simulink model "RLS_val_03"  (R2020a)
settings: Solver=ode45  StartTime=0.0  StopTime=1000  RelTol=1e-3  EnableMultiTasking=on
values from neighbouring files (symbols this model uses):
  Ts = 0.05    [init_model.m]
libraries: ctrlSharedLib x2

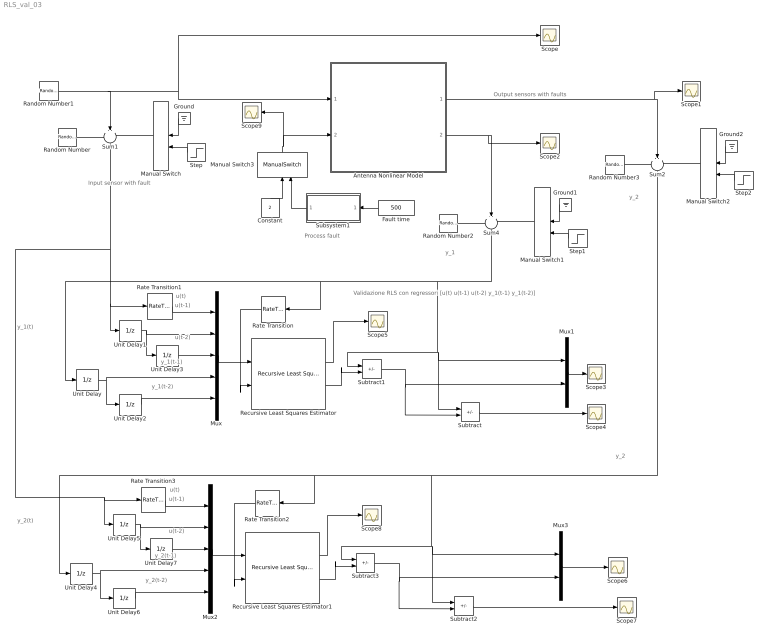
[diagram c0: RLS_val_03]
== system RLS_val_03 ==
  note: Validazione RLS con regressori [u(t) u(t-1) u(t-2) y_1(t-1) y_1(t-2)]
  note: y_1(t)
  note: y_1(t-1)
  note: y_2
  note: y_1
  note: u(t)
  note: Output sensors with faults
  note: Process fault
  note: Input sensor with fault
  note: u(t-1)
  note: y_1(t-2)
  note: u(t-2)
  note: u(t-1)
  note: y_2(t)
  note: y_2(t-1)
  note: y_2
  note: y_2(t-2)
  note: u(t-2)
  note: u(t)
  Antenna Nonlinear Model : Subsystem
  Constant : Constant  Value=2
  Fault time : Constant  Value=500
  Ground : Ground
  Ground1 : Ground
  Ground2 : Ground
  Manual Switch{,1..3} (4 alike) : ManualSwitch
  Mux : Mux  Inputs=5
  Mux1 : Mux  Inputs=2
  Mux2 : Mux  Inputs=5
  Mux3 : Mux  Inputs=2
  Random Number : RandomNumber  Variance=0.0001  Seed=1  SampleTime=Ts
  Random Number1 : RandomNumber  Variance=0.1  SampleTime=10
  Random Number2 : RandomNumber  Variance=0.00001  Seed=2  SampleTime=Ts
  Random Number3 : RandomNumber  Variance=0.00001  Seed=3  SampleTime=Ts
  Rate Transition{,1..3} (4 alike) : RateTransition  OutPortSampleTime=Ts
  Recursive Least Squares Estimator : ctrlSharedLib/Recursive Least Squares Estimator  InitialEstimateSource=None  InitialParameterData=5  P0=1e4  InitialRegressors=0  InitialOutputs=0  History=Infinite  WindowLength=200  EstimationMethod=Forgetting Factor  AdaptationParameter=1  HasTimeVaryingAdaptationParameter=off  NormalizationBias=eps  OutputError=on  OutputP=off  AddEnablePort=off  InputProcessing=Sample-based  Ts=Ts
  Recursive Least Squares Estimator1 : ctrlSharedLib/Recursive Least Squares Estimator  InitialEstimateSource=None  InitialParameterData=5  P0=1e4  InitialRegressors=0  InitialOutputs=0  History=Infinite  WindowLength=200  EstimationMethod=Forgetting Factor  AdaptationParameter=1  HasTimeVaryingAdaptationParameter=off  NormalizationBias=eps  OutputError=on  OutputP=off  AddEnablePort=off  InputProcessing=Sample-based  Ts=Ts
  Scope{,1..9} (10 alike) : Scope
  Step : Step  Time=500  SampleTime=0
  Step1 : Step  Time=1500  SampleTime=0
  Step2 : Step  Time=500  SampleTime=0
  Subsystem1 : Subsystem
  Subtract{,1..3} (4 alike) : Sum  Inputs=+-
  Sum1 : Sum  Inputs=+++  SaturateOnIntegerOverflow=on
  Sum2 : Sum  Inputs=+++  SaturateOnIntegerOverflow=on
  Sum4 : Sum  Inputs=+++  SaturateOnIntegerOverflow=on
  Unit Delay{,1..7} (8 alike) : UnitDelay  SampleTime=Ts  HasFrameUpgradeWarning=on
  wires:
  Random Number1/1 -> Scope/1, Antenna Nonlinear Model/1(force), Sum1/2
  Random Number/1 -> Sum1/1
  Manual Switch/1 -> Sum1/3
  Ground/1 -> Manual Switch/1
  Step/1 -> Manual Switch/2
  Random Number2/1 -> Sum4/1
  Ground1/1 -> Manual Switch1/1
  Manual Switch1/1 -> Sum4/3
  Step1/1 -> Manual Switch1/2
  Antenna Nonlinear Model/2(velocity) -> Sum4/2, Scope2/1
  Random Number3/1 -> Sum2/1
  Ground2/1 -> Manual Switch2/1
  Manual Switch2/1 -> Sum2/3
  Step2/1 -> Manual Switch2/2
  Antenna Nonlinear Model/1(angle) -> Sum2/2, Scope1/1
  Fault time/1 -> Subsystem1/1(Fault time)
  Subsystem1/1(Fault) -> Manual Switch3/2
  Manual Switch3/1 -> Scope9/1, Antenna Nonlinear Model/2(drag)
  Constant/1 -> Manual Switch3/1
  Mux/1 -> Recursive Least Squares Estimator/1
  Unit Delay/1 -> Mux/4, Unit Delay2/1
  Unit Delay1/1 -> Unit Delay3/1, Mux/2
  Unit Delay3/1 -> Mux/3
  Unit Delay2/1 -> Mux/5
  Subtract1/1 -> Subtract/2, Mux1/2
  Sum4/1 -> Subtract/1, Mux1/1, Subtract1/1, Rate Transition/1, Unit Delay/1
  Subtract/1 -> Scope4/1
  Mux1/1 -> Scope3/1
  Rate Transition/1 -> Recursive Least Squares Estimator/2
  Recursive Least Squares Estimator/2 -> Subtract1/2
  Recursive Least Squares Estimator/1 -> Scope5/1
  Rate Transition1/1 -> Mux/1
  Subtract3/1 -> Subtract2/2, Mux3/2
  Mux2/1 -> Recursive Least Squares Estimator1/1
  Rate Transition2/1 -> Recursive Least Squares Estimator1/2
  Rate Transition3/1 -> Mux2/1
  Recursive Least Squares Estimator1/1 -> Scope8/1
  Subtract2/1 -> Scope7/1
  Mux3/1 -> Scope6/1
  Unit Delay6/1 -> Mux2/5
  Unit Delay7/1 -> Mux2/3
  Unit Delay5/1 -> Unit Delay7/1, Mux2/2
  Unit Delay4/1 -> Mux2/4, Unit Delay6/1
  Recursive Least Squares Estimator1/2 -> Subtract3/2
  Sum2/1 -> Subtract2/1, Mux3/1, Subtract3/1, Rate Transition2/1, Unit Delay4/1
  Sum1/1 -> Unit Delay5/1, Rate Transition3/1, Unit Delay1/1, Rate Transition1/1

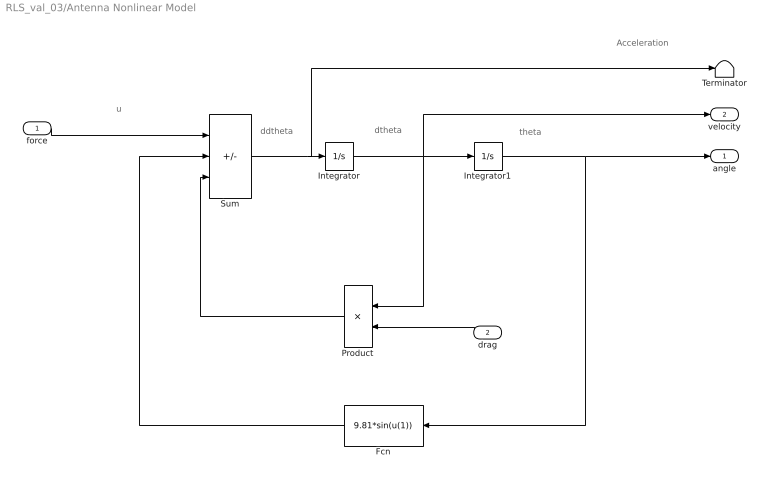
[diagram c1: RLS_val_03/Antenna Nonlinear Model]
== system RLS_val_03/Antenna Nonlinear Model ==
  note: Acceleration
  note: ddtheta
  note: dtheta
  note: theta
  note: u
  force : Inport
  drag : Inport  Port=2
  Fcn : Fcn  Expr=9.81*sin(u(1))
  Integrator : Integrator
  Integrator1 : Integrator  InitialCondition=(pi/180)*90
  Product : Product
  Sum : Sum  Inputs=+--  SaturateOnIntegerOverflow=on
  Terminator : Terminator
  angle : Outport
  velocity : Outport  Port=2
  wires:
  Sum/1 -> Terminator/1, Integrator/1
  Integrator/1 -> Product/1, Integrator1/1, velocity/1
  Integrator1/1 -> angle/1, Fcn/1
  Fcn/1 -> Sum/2
  Product/1 -> Sum/3
  force/1 -> Sum/1
  drag/1 -> Product/2

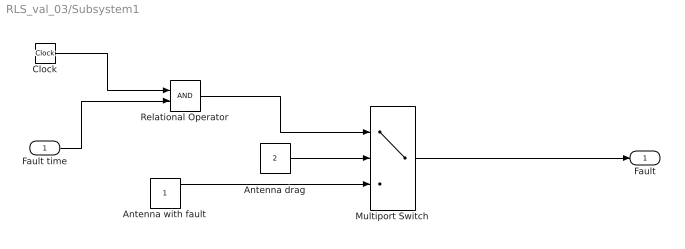
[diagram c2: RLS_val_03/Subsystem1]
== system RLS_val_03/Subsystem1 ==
  Fault time : Inport
  Antenna drag : Constant  Value=2
  Antenna with fault : Constant
  Clock : Clock
  Multiport Switch : MultiPortSwitch  DataPortOrder=Zero-based contiguous  Inputs=2  zeroidx=on
  Relational Operator : RelationalOperator  OutDataTypeStr=boolean  RndMeth=Simplest
  Fault : Outport
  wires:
  Clock/1 -> Relational Operator/1
  Fault time/1 -> Relational Operator/2
  Antenna drag/1 -> Multiport Switch/2
  Relational Operator/1 -> Multiport Switch/1
  Multiport Switch/1 -> Fault/1
  Antenna with fault/1 -> Multiport Switch/3
